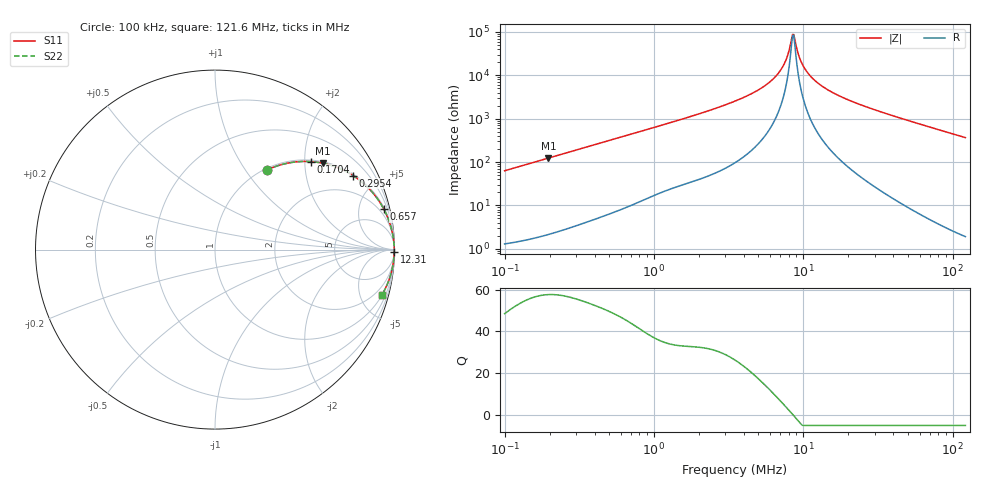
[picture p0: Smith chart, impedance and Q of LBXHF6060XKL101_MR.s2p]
! LBXHF6060XKL101_MR  S-PARAMETER MODEL  ( General Type )
! Model Generated by TAIYO YUDEN Corporation (http://www.ty-top.com)
! Version 1.0
! TAIYO YUDEN Control No. 220210
! Copyright(c) 2022 TAIYO YUDEN CO.,LTD. All Rights Reserved.
! Product Description (link to TY-COMPAS)
! https://ds.yuden.co.jp/TYCOMPAS/or/detail?pn=LBXHF6060XKL101MMR&u=M
! Products Name : Inductors
! Characteristics :
!  Inductance : 100 uH , SRF(min) : 6.5 MHz , DC Resistance(max) : 0.66 Ohm
!  Rated Current : Saturation :730 mA , Temp Rise : 880 mA
!  Case Size : 6.0 x 6.0 / 0.236 x 0.236 [mm/inch] , Thickness : 3 / 0.118 [mm/inch]
!  (Conditions: Temperature = 25 degC , DC Bias Current/Voltage = 0A / 0V)
! External Node Assignments :
!  1  o---GGG---o  2
! GND o---------o GND
! Frequency Range : 0.1MHz  -  121.638923MHz  [ 402 STEP ]
# MHz S RI R 50
! Freq[MHz].  S11 Real  S11 Imag  S21 Real  S21 Imag  S12 Real  S12 Imag  S22 Real  S22 Imag
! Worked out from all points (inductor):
!   401 points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, 100 kHz to 121.6 MHz, reference 50 ohm
!   read as one part in series: L = 100 uH near 103.6 kHz
!   highest Q = 57.6 at 196.4 kHz (marker M1), where L = 99.8 uH
!   self-resonance near 8.476 MHz
!   S11 on the Smith chart (normalised r, x): 100 kHz: 1.03, +1.26; 170.4 kHz: 1.04, +2.14; 295.4 kHz: 1.07, +3.70; 657 kHz: 1.18, +8.21; 12.31 MHz: open; 121.6 MHz: 1.04, -7.31
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0.1  0.2875 0.4424  0.7125 -0.4424  0.7125 -0.4424  0.2875 0.4424
0.170365  0.533 0.4902  0.467 -0.4902  0.467 -0.4902  0.533 0.4902
0.196373  0.6011 0.4811  0.3989 -0.4811  0.3989 -0.4811  0.6011 0.4811
0.295443  0.7698 0.4121  0.2302 -0.4121  0.2302 -0.4121  0.7698 0.4121
0.328662  0.8045 0.3876  0.1955 -0.3876  0.1955 -0.3876  0.8045 0.3876
0.656968  0.9395 0.2276  0.0605 -0.2276  0.0605 -0.2276  0.9395 0.2276
1.080188  0.9748 0.1434  0.0252 -0.1434  0.0252 -0.1434  0.9748 0.1434
3.550168  0.9971 0.0383  0.00295 -0.0383  0.00295 -0.0383  0.9971 0.0383
5.064104  0.9983 0.0211  0.00169 -0.0211  0.00169 -0.0211  0.9983 0.0211
6.493519  0.9987 0.0107  0.00127 -0.0107  0.00127 -0.0107  0.9987 0.0107
7.484824  0.9989 0.00515  0.00115 -0.00515  0.00115 -0.00515  0.9989 0.00515
7.894409  0.9989 0.00308  0.00112 -0.00308  0.00112 -0.00308  0.9989 0.00308
8.326408  0.9989 0.00103  0.0011 -0.00103  0.0011 -0.00103  0.9989 0.00103
8.475598  0.9989 0.000343  0.0011 -0.000343  0.0011 -0.000343  0.9989 0.000343
8.782046  0.9989 -0.00103  0.00109 0.00103  0.00109 0.00103  0.9989 -0.00103
9.428583  0.9989 -0.00377  0.0011 0.00377  0.0011 0.00377  0.9989 -0.00377
9.944535  0.9989 -0.00584  0.00111 0.00584  0.00111 0.00584  0.9989 -0.00584
11.46267  0.9988 -0.0115  0.00119 0.0115  0.00119 0.0115  0.9988 -0.0115
12.30656  0.9987 -0.0143  0.00126 0.0143  0.00126 0.0143  0.9987 -0.0143
18.5152  0.9979 -0.0328  0.00212 0.0328  0.00212 0.0328  0.9979 -0.0328
37.67347  0.9925 -0.0801  0.00752 0.0801  0.00752 0.0801  0.9925 -0.0801
121.6389  0.9292 -0.2538  0.0708 0.2538  0.0708 0.2538  0.9292 -0.2538
